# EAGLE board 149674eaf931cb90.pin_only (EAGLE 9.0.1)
REV: B

Size 68.58 x 53.34 mm. Coordinates in mm from the lower left corner, seen from the top.
Copper layers (1*16): Top 0.035mm / dielectric 1.5mm / Bottom 0.035mm
Design rules "adafruit *": minimum track width 8mil, minimum drill 15.5mil, track to track 8mil, track to pad 8mil, pad to pad 8mil, via to via 8mil, smd to smd 8mil, copper to edge 10mil, drill to drill 8mil, minimum pad ring 10mil, minimum via ring 8mil, stop-mask expansion 2mil, vias tented up to drill 20mil, thermal gap 10mil
Net classes: 1 power: width 0.305 mm

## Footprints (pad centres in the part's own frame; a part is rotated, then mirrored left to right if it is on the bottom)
SOLDERJUMPER_ARROW_NOPASTE = smd 0.762 x 1.524: 1 -1.016,0; 2 1.016,0
1X06_ROUND = drill 1 pad 1.676: 1 -6.35,0; 2 -3.81,0; 3 -1.27,0; 4 1.27,0; 5 3.81,0; 6 6.35,0
EVQ-Q2_SMALLER = smd 2 x 1.2: A -3.1,-2; A' 3.1,-2; B -3.1,2; B' 3.1,2
0805-NO = smd 1.24 x 1.5: 1 -0.95,0; 2 0.95,0
1X08_ROUND = drill 1 pad 1.676: 1 -8.89,0; 2 -6.35,0; 3 -3.81,0; 4 -1.27,0; 5 1.27,0; 6 3.81,0; 7 6.35,0; 8 8.89,0
FIDUCIAL_1MM = smd 1 x 1: 1 0,0
QFN24_4MM = smd 0.8 x 0.28: 1 -2,1.25; 2 -2,0.75; 3 -2,0.25; 4 -2,-0.25; 5 -2,-0.75; 6 -2,-1.25; 13 2,-1.25; 14 2,-0.75; 15 2,-0.25; 16 2,0.25; 17 2,0.75; 18 2,1.25 | smd 0.28 x 0.8: 7 -1.25,-2; 8 -0.75,-2; 9 -0.25,-2; 10 0.25,-2; 11 0.75,-2; 12 1.25,-2; 19 1.25,2; 20 0.75,2; 21 0.25,2; 22 -0.25,2; 23 -0.75,2; 24 -1.25,2 | smd 1.778 x 1.778: THERM 0,0
SOT23-5L = smd 0.55 x 1.2: 1 -0.95,-1.3; 2 0,-1.3; 3 0.95,-1.3; 4 0.95,1.3; 5 -0.95,1.3
1X10_ROUND = drill 1 pad 1.676: 1 -11.43,0; 2 -8.89,0; 3 -6.35,0; 4 -3.81,0; 5 -1.27,0; 6 1.27,0; 7 3.81,0; 8 6.35,0; 9 8.89,0; 10 11.43,0
ARDUINOR3_ICSP = drill 1 pad 1.676 octagon: 3V 35.56,2.54; 5V 38.1,2.54; A0 50.8,2.54; A1 53.34,2.54; A2 55.88,2.54; A3 58.42,2.54; A4 60.96,2.54; A5 63.5,2.54; AREF 23.876,50.8; D0 63.5,50.8; D1 60.96,50.8; D2 58.42,50.8; D3 55.88,50.8; D4 53.34,50.8; D5 50.8,50.8; D6 48.26,50.8; D7 45.72,50.8; D8 41.656,50.8; D9 39.116,50.8; D10 36.576,50.8; D11 34.036,50.8; D12 31.496,50.8; D13 28.956,50.8; GND 26.416,50.8; GND@1 43.18,2.54; GND@2 40.64,2.54; IOREF 30.48,2.54; RESERVED 27.94,2.54; RESET 33.02,2.54; SCL 18.796,50.8; SDA 21.336,50.8; VIN 45.72,2.54 | drill 1 pad 1.778 octagon: 5V_ICSP 66.167,30.48; GND@3 66.167,25.4; MOSI 66.167,27.94; RESET_ICSP 63.627,25.4; SCK 63.627,27.94 | drill 1 pad 1.778 square: MISO 63.627,30.48
SOT23-WIDE = smd 1 x 1.2: 1 -0.95,-1; 2 0.95,-1; 3 0,1
SOT363 = smd 0.5 x 0.5: 1 -0.75,-0.9; 3 0.75,-0.9; 4 0.75,0.9; 6 -0.75,0.9 | smd 0.4 x 0.5: 2 0,-0.9; 5 0,0.9
RESPACK_4X0603_NO = smd 0.45 x 0.9: 1 -1.3,-0.85; 2 -0.4,-0.85; 3 0.4,-0.85; 4 1.3,-0.85; 5 1.3,0.85; 6 0.4,0.85; 7 -0.4,0.85; 8 -1.3,0.85
SKQUBAE010 = smd 1.5 x 1.4: 1 -5.2,3.25; 2 -5.2,-0.45; 3 -5.2,-3.25; 4 5.2,-3.25; 5 5.2,-0.45; 6 5.2,3.25
TESTPOINT_ROUND_2MM = smd 2 x 2: P$1 0,0
TSSOP16 = smd 0.305 x 0.991: 1 -2.275,-2.918; 2 -1.625,-2.918; 3 -0.975,-2.918; 4 -0.325,-2.918; 5 0.325,-2.918; 6 0.975,-2.918; 7 1.625,-2.918; 8 2.275,-2.918; 9 2.275,2.918; 10 1.625,2.918; 11 0.975,2.918; 12 0.325,2.918; 13 -0.325,2.918; 14 -0.975,2.918; 15 -1.625,2.918; 16 -2.275,2.918
JD-T1800 = smd 0.5 x 2: 1 5.2,-13.1; 2 4.4,-13.1; 3 3.6,-13.1; 4 2.8,-13.1; 5 2,-13.1; 6 1.2,-13.1; 7 0.4,-13.1; 8 -0.4,-13.1; 9 -1.2,-13.1; 10 -2,-13.1; 11 -2.8,-13.1; 12 -3.6,-13.1; 13 -4.4,-13.1; 14 -5.2,-13.1 | hole 0.6: -12.8,-16.9; 7.65,-16.9
MICROSD = smd 0.7 x 1.5: 1 9,-10.64; 2 7.9,-10.24; 3 6.8,-10.64; 4 5.7,-11.04; 5 4.6,-10.64; 6 3.5,-11.04; 7 2.4,-10.64; 8 1.3,-10.64 | smd 1.8 x 1.4: CD1 2,-0.44; CD2 8,-0.44 | smd 1.4 x 1.9: MT1 0.4,-13.54; MT2 13.6,-14.44

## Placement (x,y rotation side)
AD0  [SOLDERJUMPER_ARROW_NOPASTE]  62.1,36.96 0 bottom
AD1  [SOLDERJUMPER_ARROW_NOPASTE]  62.1,39.88 0 bottom
ANALOGS  [1X06_ROUND]  57.15,5.84 180 top
BTN1  EVQQ  [EVQ-Q2_SMALLER]  3.81,5.08 90 top
BTN2  EVQQ  [EVQ-Q2_SMALLER]  12.7,5.08 90 top
BTN3  EVQQ  [EVQ-Q2_SMALLER]  21.59,5.08 90 top
C1  10uF  [0805-NO]  39.37,8.89 0 top
C2  10uF  [0805-NO]  32.26,8.89 90 top
C3  0.1uF  [0805-NO]  49.28,12.19 180 top
C4  0.1uF  [0805-NO]  30.23,8.89 90 top
DIGITALS  [1X08_ROUND]  54.61,46.99 0 top
DIGITALS1  [1X08_ROUND]  36.83,5.84 180 top
FID1  FIDUCIAL_1MM  [FIDUCIAL_1MM]  3.17,43.31 0 top
FID3  FIDUCIAL_1MM  [FIDUCIAL_1MM]  43.56,15.49 0 top
IC1  ATSAMD09D14A-MU  [QFN24_4MM]  60.45,38.35 90 top
IC2  AP2112K-3.3  [SOT23-5L]  35.56,8.89 90 top
JP1  [1X10_ROUND]  30.23,46.99 0 top
M1  ARDUINO_R3_ICSP  [ARDUINOR3_ICSP]  0,0 0 top
Q2  BSS138  [SOT23-WIDE]  49.15,17.78 0 top
Q3  BSS138  [SOT363]  63.12,43.94 90 top
R1  22 ohm  [0805-NO]  49.15,21.08 0 top
R2  10K  [0805-NO]  48.39,43.94 180 top
R5  1K  [0805-NO]  55.5,36.32 270 top
R8  10K  [RESPACK_4X0603_NO]  56.77,43.18 180 top
R9  10K  [0805-NO]  49.28,14.73 0 top
RESET  EVQQ  [EVQ-Q2_SMALLER]  5.84,49.15 180 top
SW1  NAVSWITCHSKQUABAUE010  [SKQUBAE010]  53.72,29.21 0 top
TP1  [TESTPOINT_ROUND_2MM]  55.37,39.37 0 bottom
TP2  [TESTPOINT_ROUND_2MM]  55.37,36.07 0 bottom
U1  74HC4050  [TSSOP16]  50.55,40.13 270 top
U$1  DISP_LCD_JDT1800  [JD-T1800]  23.24,28.07 90 top
U$3  MICROSD  [MICROSD]  51.82,8.38 90 top
U$5  [ADAFRUIT_TEXT_30MM]  40.39,31.5 0 bottom
U$7  [ADAFRUIT_5MM]  11.56,46.99 0 top
U$8  [SEESAW_LOGO]  31.5,27.43 0 bottom
U$9  [PCBFEAT-REV-040]  49.28,7.87 0 top

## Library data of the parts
AD0 AD1 FID1 FID3 = microbuilder; BOM: EXCLUDE
ANALOGS BTN1-BTN3 C1-C4 DIGITALS DIGITALS1 IC1 JP1 Q2 Q3 R1 R2 R5 R8 R9 RESET SW1 TP1 TP2 U1 U$1 U$5 U$7 U$9 = microbuilder
IC2 M1 U$3 = adafruit
U$8 = silks

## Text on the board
tPlace: Reset | A | B | C | 1.8" TFT / Shield
bPlace: DC | TCS | CCS | AD1 | AD0 | Adafruit 1.8" TFT Shield / with MicroSD Card / 5-Way Nav + 3 Buttons | buttons/nav and backlight controlled by seesaw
